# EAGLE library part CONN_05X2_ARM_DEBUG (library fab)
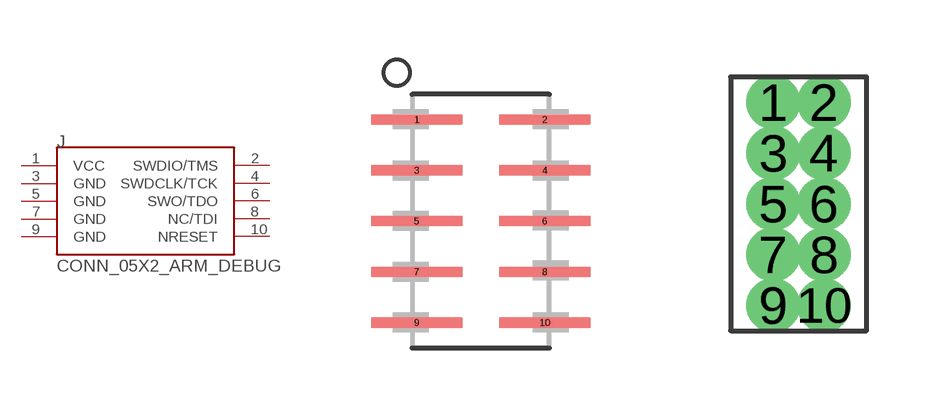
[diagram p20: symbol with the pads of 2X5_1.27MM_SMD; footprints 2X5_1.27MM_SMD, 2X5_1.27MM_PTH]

Designator prefix J

## CONN_05X2_ARM_DEBUGSMD (PACKAGE: 2x5_1.27MM_SMD)  [2X5_1.27MM_SMD]
1  VCC
2  SWDIO/TMS
3  GND
4  SWDCLK/TCK
5  GND
6  SWO/TDO
7  GND
8  NC/TDI
9  GND
10  NRESET

## CONN_05X2_ARM_DEBUGPTH (PACKAGE: 2x5_1.27MM_PTH)  [2X5_1.27MM_PTH]
Pads as for 2X5_1.27MM_SMD

## CONN_05X2_ARM_DEBUGTDC2050-IDC (PACKAGE: TC2050-IDC)  [TC2050-IDC]
Pads as for 2X5_1.27MM_SMD

## Footprint 2X5_1.27MM_SMD (pad centres in mm)
smd 2.286 x 0.254: 1 -1.6,2.54; 2 1.6,2.54; 3 -1.6,1.27; 4 1.6,1.27; 5 -1.6,0; 6 1.6,0; 7 -1.6,-1.27; 8 1.6,-1.27; 9 -1.6,-2.54; 10 1.6,-2.54

## Footprint 2X5_1.27MM_PTH (pad centres in mm)
drill 0.838 pad 1.016: 1 -0.635,2.54; 2 0.635,2.54; 3 -0.635,1.27; 4 0.635,1.27; 5 -0.635,0; 6 0.635,0; 7 -0.635,-1.27; 8 0.635,-1.27; 9 -0.635,-2.54; 10 0.635,-2.54

## Footprint TC2050-IDC (pad centres in mm)
smd 0.787 x 0.787: 1 1.27,-0.635; 2 2.54,-0.635; 3 3.81,-0.635; 4 5.08,-0.635; 5 6.35,-0.635; 6 6.35,0.635; 7 5.08,0.635; 8 3.81,0.635; 9 2.54,0.635; 10 1.27,0.635
hole 0.991 at 0,0
hole 0.991 at 7.62,1.016
hole 0.991 at 7.62,-1.016
hole 2.375 at 0,2.54
hole 2.375 at 5.715,2.54
hole 2.375 at 0,-2.54
hole 2.375 at 5.715,-2.54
